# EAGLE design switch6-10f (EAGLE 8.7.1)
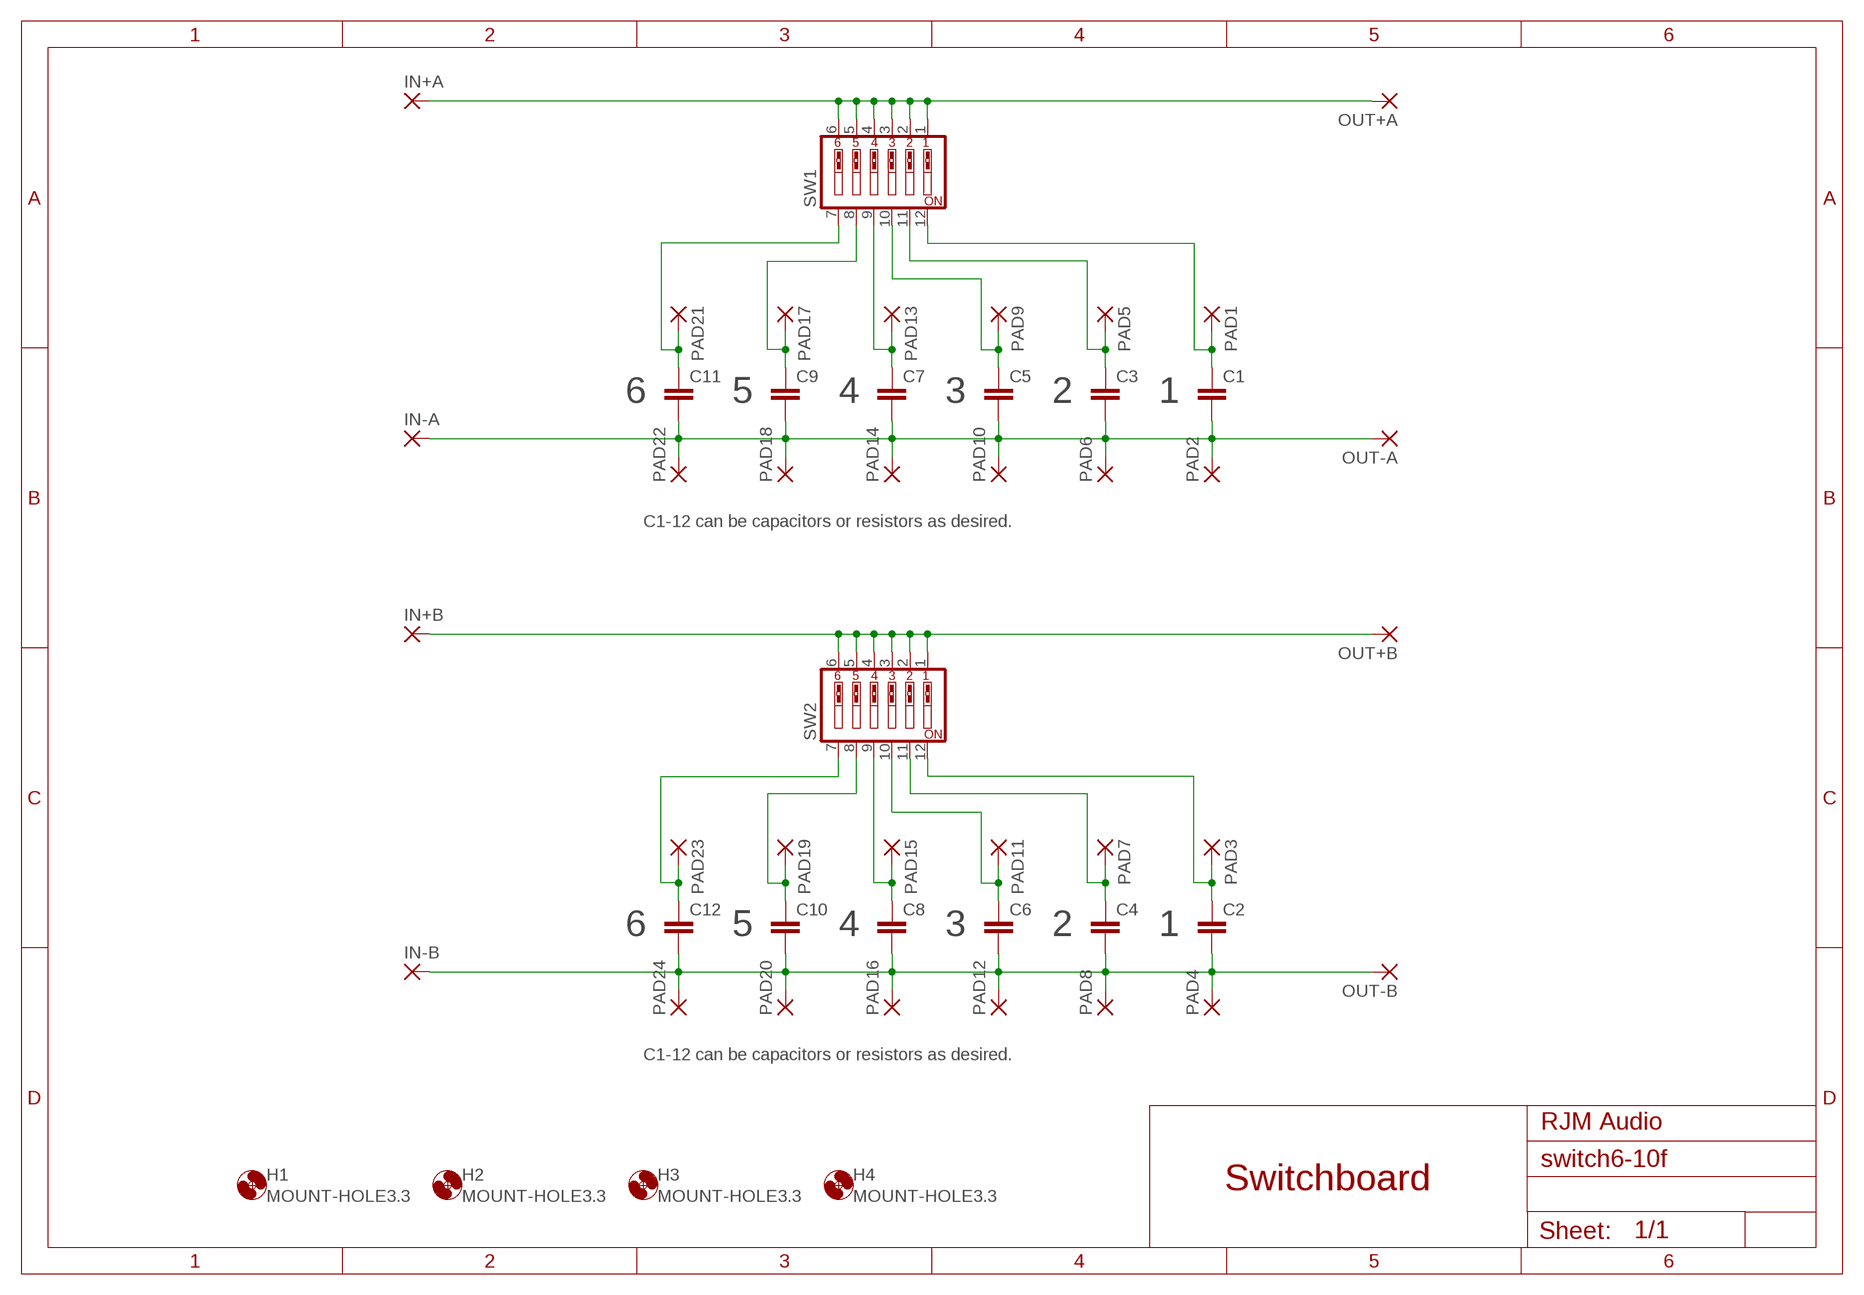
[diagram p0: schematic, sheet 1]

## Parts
C1  C-EU050-045X075  [C050-045X075]
C2  C-EU050-045X075  [C050-045X075]
C3  C-EU050-045X075  [C050-045X075]
C4  C-EU050-045X075  [C050-045X075]
C5  C-EU050-045X075  [C050-045X075]
C6  C-EU050-045X075  [C050-045X075]
C7  C-EU050-045X075  [C050-045X075]
C8  C-EU050-045X075  [C050-045X075]
C9  C-EU050-045X075  [C050-045X075]
C10  C-EU050-045X075  [C050-045X075]
C11  C-EU050-045X075  [C050-045X075]
C12  C-EU050-045X075  [C050-045X075]
H1  MOUNT-HOLE3.3  [3,3]
H2  MOUNT-HOLE3.3  [3,3]
H3  MOUNT-HOLE3.3  [3,3]
H4  MOUNT-HOLE3.3  [3,3]
IN+A  3,17/1,3  [3,17/1,3]
IN+B  3,17/1,3  [3,17/1,3]
IN-A  3,17/1,3  [3,17/1,3]
IN-B  3,17/1,3  [3,17/1,3]
OUT+A  3,17/1,3  [3,17/1,3]
OUT+B  3,17/1,3  [3,17/1,3]
OUT-A  3,17/1,3  [3,17/1,3]
OUT-B  3,17/1,3  [3,17/1,3]
PAD1  1,6/0,8  [1,6/0,8]
PAD2  1,6/0,8  [1,6/0,8]
PAD3  1,6/0,8  [1,6/0,8]
PAD4  1,6/0,8  [1,6/0,8]
PAD5  1,6/0,8  [1,6/0,8]
PAD6  1,6/0,8  [1,6/0,8]
PAD7  1,6/0,8  [1,6/0,8]
PAD8  1,6/0,8  [1,6/0,8]
PAD9  1,6/0,8  [1,6/0,8]
PAD10  1,6/0,8  [1,6/0,8]
PAD11  1,6/0,8  [1,6/0,8]
PAD12  1,6/0,8  [1,6/0,8]
PAD13  1,6/0,8  [1,6/0,8]
PAD14  1,6/0,8  [1,6/0,8]
PAD15  1,6/0,8  [1,6/0,8]
PAD16  1,6/0,8  [1,6/0,8]
PAD17  1,6/0,8  [1,6/0,8]
PAD18  1,6/0,8  [1,6/0,8]
PAD19  1,6/0,8  [1,6/0,8]
PAD20  1,6/0,8  [1,6/0,8]
PAD21  1,6/0,8  [1,6/0,8]
PAD22  1,6/0,8  [1,6/0,8]
PAD23  1,6/0,8  [1,6/0,8]
PAD24  1,6/0,8  [1,6/0,8]
SW1  SW_DIP-6  [EDG-06]
SW2  SW_DIP-6  [EDG-06]

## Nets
GNDL: C2.2 C4.2 C6.2 C8.2 C10.2 C12.2 IN-B.1(P) OUT-B.1(P) PAD4.1(P) PAD8.1(P) PAD12.1(P) PAD16.1(P) PAD20.1(P) PAD24.1(P)
GNDR: C1.2 C3.2 C5.2 C7.2 C9.2 C11.2 IN-A.1(P) OUT-A.1(P) PAD2.1(P) PAD6.1(P) PAD10.1(P) PAD14.1(P) PAD18.1(P) PAD22.1(P)
L+: IN+B.1(P) OUT+B.1(P) SW2.1 SW2.2 SW2.3 SW2.4 SW2.5 SW2.6
N$2: C6.1 PAD11.1(P) SW2.10
N$3: C1.1 PAD1.1(P) SW1.12
N$6: C2.1 PAD3.1(P) SW2.12
N$15: C4.1 PAD7.1(P) SW2.11
N$16: C3.1 PAD5.1(P) SW1.11
N$18: C5.1 PAD9.1(P) SW1.10
N$19: C8.1 PAD15.1(P) SW2.9
N$20: C7.1 PAD13.1(P) SW1.9
N$21: C10.1 PAD19.1(P) SW2.8
N$22: C9.1 PAD17.1(P) SW1.8
N$23: C12.1 PAD23.1(P) SW2.7
N$24: C11.1 PAD21.1(P) SW1.7
R+: IN+A.1(P) OUT+A.1(P) SW1.1 SW1.2 SW1.3 SW1.4 SW1.5 SW1.6

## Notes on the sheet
- 6 | 5 | 4 | 3 | 2 | 1
- C1-12 can be capacitors or resistors as desired.
- 6 | 5 | 4 | 3 | 2 | 1
- C1-12 can be capacitors or resistors as desired.
- RJM Audio
- Switchboard

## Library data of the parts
C1-C12 = resistor:C-EU: CAPACITOR, European symbol
H1-H4 = holes:MOUNT-HOLE: MOUNTING HOLE with drill center marker
IN+A IN+B IN-A IN-B OUT+A OUT+B OUT-A OUT-B = wirepad:3,17/1,3: THROUGH-HOLE PAD
PAD1-PAD24 = wirepad:1,6/0,8: THROUGH-HOLE PAD
SW1 SW2 = special:SW_DIP-6: DIP SWITCH

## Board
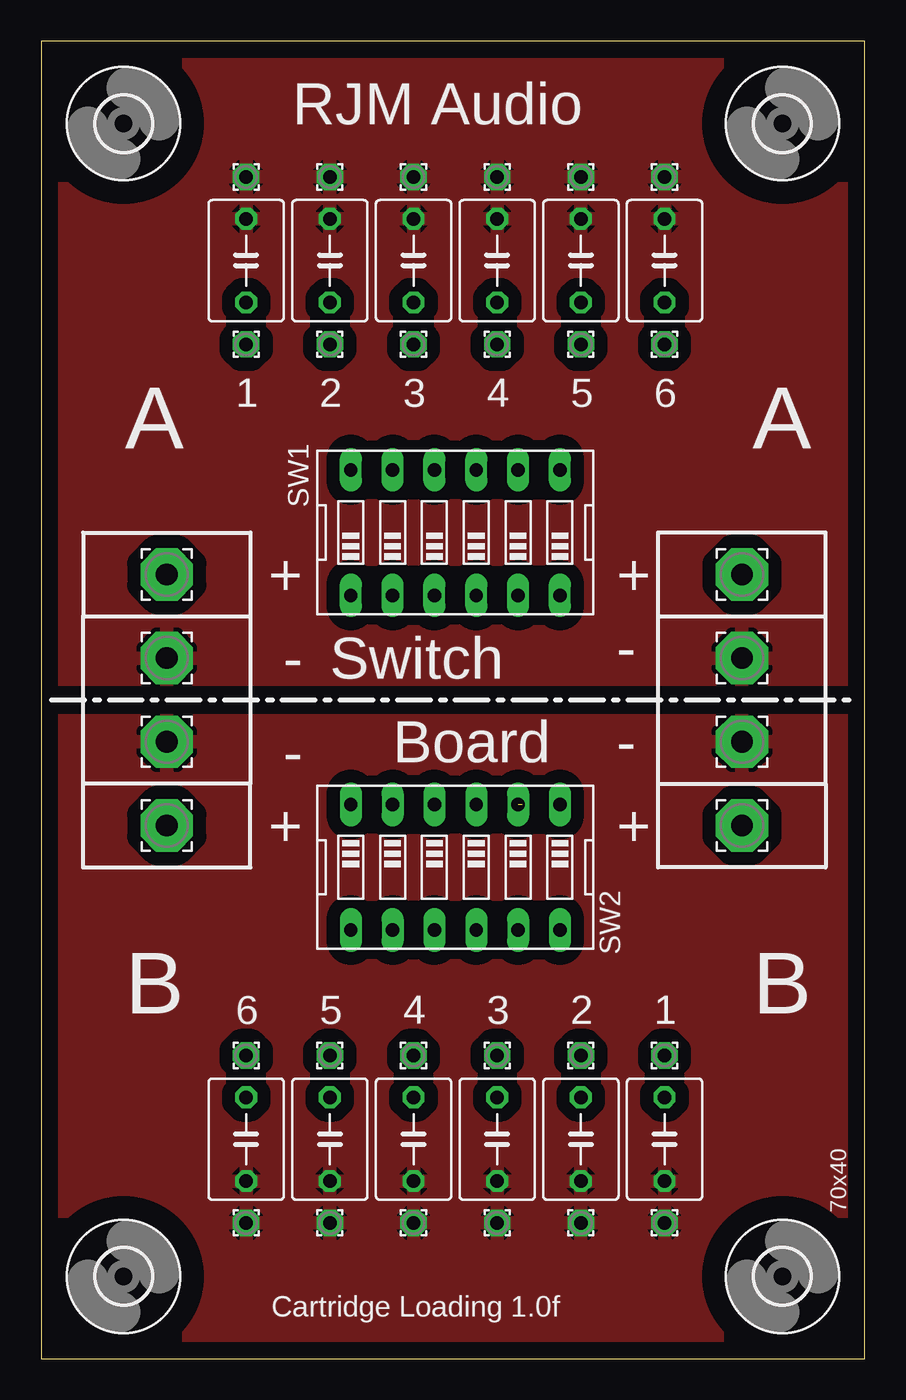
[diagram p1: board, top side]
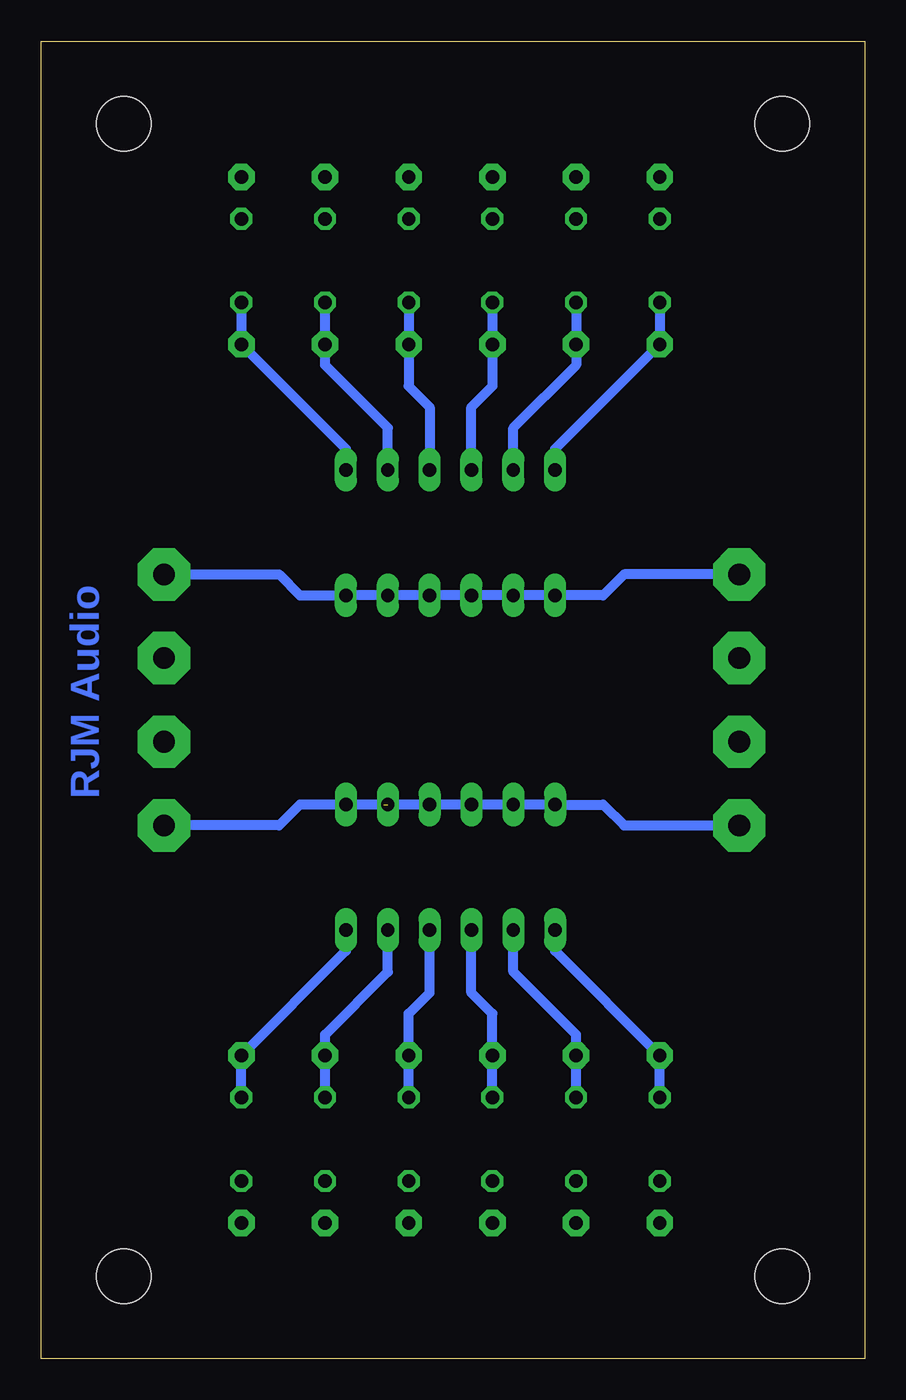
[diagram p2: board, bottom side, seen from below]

Size 50 x 80 mm. Coordinates in mm from the lower left corner, seen from the top.
Outline: 0,0 50,0 50,80 0,80 0,0
Copper layers (1*16): Top 0.035mm / dielectric 1.5mm / Bottom 0.035mm
Design rules "default": minimum track width 10mil, minimum drill 24mil, track to track 8mil, track to pad 8mil, pad to pad 8mil, via to via 8mil, smd to smd 8mil, copper to edge 40mil, drill to drill 8mil, minimum pad ring 10mil, minimum via ring 8mil, stop-mask expansion 4mil, vias tented up to drill 0mil, thermal gap 10mil

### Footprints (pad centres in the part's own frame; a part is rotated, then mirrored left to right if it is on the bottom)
C050-045X075 = drill 0.813 octagon: 1 -2.54,0; 2 2.54,0
3,3 = hole 3.3: 0,0
3,17/1,3 = drill 1.321 pad 3.175 octagon: 1 0,0
1,6/0,8 = drill 0.813 pad 1.6 octagon: 1 0,0
EDG-06 = drill 0.813 long: 1 -6.35,-3.81; 2 -3.81,-3.81; 3 -1.27,-3.81; 4 1.27,-3.81; 5 3.81,-3.81; 6 6.35,-3.81; 7 6.35,3.81; 8 3.81,3.81; 9 1.27,3.81; 10 -1.27,3.81; 11 -3.81,3.81; 12 -6.35,3.81

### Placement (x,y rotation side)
C1  12.45,66.67 90 top
C2  37.85,13.34 270 top
C3  17.53,66.67 90 top
C4  32.77,13.34 270 top
C5  22.61,66.67 90 top
C6  27.69,13.34 270 top
C7  27.69,66.67 90 top
C8  22.61,13.34 270 top
C9  32.77,66.67 90 top
C10  17.53,13.34 270 top
C11  37.85,66.67 90 top
C12  12.45,13.34 270 top
H1  5,75 0 top
H2  45,75 0 top
H3  5,5 0 top
H4  45,5 0 top
IN+A  7.62,47.62 0 top
IN+B  7.62,32.39 0 top
IN-A  7.62,42.55 0 top
IN-B  7.62,37.47 0 top
OUT+A  42.55,47.62 0 top
OUT+B  42.55,32.39 0 top
OUT-A  42.55,42.55 0 top
OUT-B  42.55,37.47 0 top
PAD1  12.45,61.59 0 top
PAD2  12.45,71.75 0 top
PAD3  37.85,18.41 0 top
PAD4  37.85,8.26 0 top
PAD5  17.53,61.59 0 top
PAD6  17.53,71.75 0 top
PAD7  32.77,18.41 0 top
PAD8  32.77,8.26 0 top
PAD9  22.61,61.59 0 top
PAD10  22.61,71.75 0 top
PAD11  27.69,18.41 0 top
PAD12  27.69,8.26 0 top
PAD13  27.69,61.59 0 top
PAD14  27.69,71.75 0 top
PAD15  22.61,18.41 0 top
PAD16  22.61,8.26 0 top
PAD17  32.77,61.59 0 top
PAD18  32.77,71.75 0 top
PAD19  17.53,18.41 0 top
PAD20  17.53,8.26 0 top
PAD21  37.85,61.59 0 top
PAD22  37.85,71.75 0 top
PAD23  12.45,18.41 0 top
PAD24  12.45,8.26 0 top
SW1  25.15,50.16 0 top
SW2  25.15,29.84 180 top

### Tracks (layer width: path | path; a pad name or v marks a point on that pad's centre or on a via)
GNDL
  pour Top (isolate 0.813): 0,38.73 0,-0.64 50.16,-0.64 50.16,38.73
GNDR
  pour Top (isolate 0.813): 0,80.01 50.16,80.01 50.16,41.27 0,41.27
L+  (1 unrouted)
  Bottom 0.61: 29.21,33.66 SW2.3 SW2.4 SW2.5 SW2.6 15.88,33.66 14.61,32.39 IN+B.1 | SW2.2 SW2.1 34.29,33.66 35.56,32.39 OUT+B.1
N$2
  Bottom 0.61: SW2.10 26.42,22.22 27.69,20.95 PAD11.1 C6.1
N$3
  Bottom 0.61: C1.1 PAD1.1 18.8,55.25 SW1.12
N$6
  Bottom 0.61: SW2.12 31.5,24.76 PAD3.1 C2.1
N$15
  Bottom 0.61: SW2.11 28.96,23.49 32.77,19.68 PAD7.1 C4.1
N$16
  Bottom 0.61: SW1.11 21.34,56.52 17.53,60.33 PAD5.1 C3.1
N$18
  Bottom 0.61: SW1.10 23.88,57.79 22.61,59.05 PAD9.1 C5.1
N$19
  Bottom 0.61: SW2.9 23.88,22.22 22.61,20.95 PAD15.1 C8.1
N$20
  Bottom 0.61: C7.1 PAD13.1 27.69,59.05 26.42,57.79 SW1.9
N$21
  Bottom 0.61: SW2.8 21.34,23.49 17.53,19.68 PAD19.1 C10.1
N$22
  Bottom 0.61: SW1.8 28.96,56.52 32.77,60.33 PAD17.1 C9.1
N$23
  Bottom 0.61: SW2.7 18.8,24.76 PAD23.1 C12.1
N$24
  Bottom 0.61: SW1.7 31.5,55.25 PAD21.1 C11.1
R+
  Bottom 0.61: IN+A.1 14.61,47.62 15.88,46.36 SW1.1 SW1.2 SW1.3 | OUT+A.1 35.56,47.62 34.29,46.36 SW1.6 SW1.5 SW1.4 SW1.3 | 24.13,46.36 SW1.3

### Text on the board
Bottom: RJM Audio
tPlace: RJM Audio | 1 | 2 | 3 | 4 | 5 | 6 | A | A | + | + | - | - | Switch | - | Board | - | + | + | B | B | 6 | 5 | 4 | 3 | 2 | 1 | 70x40 | Cartridge Loading 1.0f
